(* Logix 5000 Rung export; software revision 16.03 *)

MODULES
   Local : vendor None type None code None
   PDPMV1_LEGACY : vendor None type None code None
END_MODULES

TYPE PDPMV1_SetSlaveAddress_In :   // Mailbox response
STRUCT
   ByteCount : INT;   // Byte count data block
   NewSlaveAddress : SINT;   // Range 1 to 125, specifies the new address of the slave.
   CurrentSlaveAddress : SINT;   // Range 1 to 125, specifies the current address of the slave.
   SlaveIdentNumber : INT;   // Ident number for the slave, which address should be altered.
   No_add_Chg : INT;   // This parameter specifies whether it is allowed to change the slave address again
   ErrorCode1_2 : INT;   // If other than 0, refer to user manual for code information
   ErrorCode3_4 : INT;   // If other than 0, refer to user manual for code information
   ReturnCode : INT;   // If other than 0, refer to user manual for code information
   FaultInformation : INT;   // If other than 0, refer to user manual for code information
   MessageDataByte : SINT[400];   // Message data byte array for user-specific data
END_STRUCT
END_TYPE

TYPE PDPMV1_Module :   // Status data
STRUCT
   Mod_scan_count : INT;   // Incremented every module scan loop
   Mod_output_update : INT;   // Incremented at every output scan
   Mod_input_update : INT;   // Incremented at every input scan
   Mod_out_MB : INT;   // Incremented at every output mailbox processing
   Mod_in_MB : INT;   // Incremented at every intput mailbox processing
   Mod_alarm_ind : INT;   // Incremented at every alarm indication
   Mod_alarm_con : INT;   // Incremented at every alarm confirmation
   Reserved1 : INT;   // Reserved
   Reserved2 : INT;   // Reserved
END_STRUCT
END_TYPE

TYPE PDPMV1_GetSlaveConfig :   // GetSlaveConfig mailobox to retrieve configuration data from specific PROFIBUS slaves
STRUCT
   Out : PDPMV1_GetSlaveConfig_Out;   // mailbox request
   In : PDPMV1_GetSlaveConfig_In;   // mailbox response
END_STRUCT
END_TYPE

TYPE PDPMV1_CRC :   // Module CRC status
STRUCT
   ProfibusCRC : DINT;   // CRC value related to the PROFIBUS configuration that was downloaded to the module
   ModuleCRC : DINT;   // CRC value related to the module configuration that was downloaded to the module
END_STRUCT
END_TYPE

TYPE PDPMV1_backplane2 :   // Stores variables used by sample ladder logic for handshaking purposes.
STRUCT
   LastRead : INT;   // Last read block index received from the module
   LastWrite : INT;   // Last write block index received from the module
   BlockIndex : INT;   // Block index of each copy of PROFIBUS input and output blocks
END_STRUCT
END_TYPE

TYPE PDPMV1_SetSlaveMode_Out :   // Mailbox Request
STRUCT
   GroupSelect : SINT;   // Range 01h to FFh (Bit Coded). This parameter determines which group to address. Refer to the user manual for examples
   SlaveAddress : SINT;   // Range 1 to 125; 127 (Multicast address).
   ControlCommand : PDPMV1_ControlCommand;   // This parameter specifies the command to send (Unsync/Sync and Unfreeze/Freeze).
END_STRUCT
END_TYPE

TYPE PDPMV1_StopSlaves_Out :   // Mailbox request
STRUCT
   SlaveNumber : SINT[126];   // Slave number designation (1-125)
END_STRUCT
END_TYPE

TYPE PDPMV1_GetSlaveConfig_Out :   // GetSlaveConfig mailbox request
STRUCT
   SlaveAddress : INT;   // Destination of slave (1-125)
END_STRUCT
END_TYPE

TYPE PDPMV1_GetSlaveDiagnostics_In :   // GetSlaveDiagnostics mailbox response
STRUCT
   SlaveAddress : INT;   // Destination of slave (1-125)
   ExtendedFaultInfo : INT;   // If other than 0, refer to user manual for code information
   FaultInformation : INT;   // If other than 0, refer to user manual for code information
   StationStatus1_2 : INT;   // Status of station types 1 and 2
   StationStatus3_4 : INT;   // Status of station types 3 and 4
   IdentNumber : INT;   // Unique ID assigned by the PROFIBUS User Organization
   ExtendedDiagnosticData : INT[200];   // Slave user-specific data. Refer to actual slave documentation for info
END_STRUCT
END_TYPE

TYPE PDPMV1_AcyclicRead :   // DPV1 acyclic read mailbox data structure
STRUCT
   Out : PDPMV1_AcyclicRead_Out;   // mailbox request
   In : PDPMV1_AcyclicRead_In;   // mailbox response
END_STRUCT
END_TYPE

TYPE PDPMV1_StartSlaves_In :   // Mailbox Response
STRUCT
   AdditionalFaultInfo : INT;   // If other than 0, refer to user manual for code information
   FaultInformation : INT;   // If other than 0, refer to user manual for code information
   SlaveNumber : SINT[126];   // Slave number designation (1-125)
END_STRUCT
END_TYPE

TYPE PDPMV1_AcyclicWrite :   // DPV1 acyclic write mailbox data structure
STRUCT
   Out : PDPMV1_AcyclicWrite_Out;   // Mailbox request
   In : PDPMV1_AcyclicWrite_In;   // Mailbox response
END_STRUCT
END_TYPE

TYPE PDPMV1_StartSlaves_Out :   // Mailbox Request
STRUCT
   SlaveNumber : SINT[126];   // Slave number designation (1-125)
END_STRUCT
END_TYPE

TYPE PDPMV1_GetSlaveDiagnostics :   // GetSlaveDiagnostics mailbox to retrieve diagnostic information from specific PROFIBUS slaves
STRUCT
   Out : PDPMV1_GetSlaveDiagnostics_Out;   // Mailbox request
   In : PDPMV1_GetSlaveDiagnostics_In;   // Mailbox response
END_STRUCT
END_TYPE

TYPE PDPMV1_backplane :   // Stores variables used by sample ladder logic for handshaking purposes.
STRUCT
   Read : INT;   // Backplane read statistics
   Write : INT;   // Backplane write statistics
   Error : INT;   // Backplane error statistics
   LastRead : INT;   // Last read block index received from the module
   LastWrite : INT;   // Last write block index received from the module
   BlockIndex : INT;   // Block index of each copy of PROFIBUS input and output blocks
END_STRUCT
END_TYPE

TYPE PDPMV1_other_status :
STRUCT
   Cfg_file_error : INT;   // Bit0 = PDPMV1.CFG, Bit 1 = WATTCP.CFG, Bit 2 = PDPMV1.DDB, Bit3=PDPMV1.XML
   R_120 : INT;   // Not Used
   R_122 : INT;   // Not Used
   R_124 : INT;   // Not Used
   R_126 : INT;   // Not Used
   R_128 : INT;   // Not Used
   R_130 : INT;   // Not Used
   R_132 : INT;   // Not Used
   R_134 : INT;   // Not Used
   R_136 : INT;   // Not Used
   R_138 : INT;   // Not Used
   R_140 : INT;   // Not Used
   R_142 : INT;   // Not Used
   R_144 : INT;   // Not Used
   In_MB_queue : INT;   // Number of messages in the input mailbox queue
   Out_MB_queue : INT;   // Number of messages in the output mailbox queue
   Alarm_MB_queue : INT;   // Number of messages in the alarm mailbox queue
   Last_out_MB : INT;   // Number of messages in the output mailbox queue
   Cur_in_MB : INT;   // Number of messages currently in the input mailbox queue
   Cur_alarm_MB : INT;   // Number of messages currently in the alarm mailbox queue
END_STRUCT
END_TYPE

TYPE PDPMV1_ControlCommand :   // Option bits for SetSlaveMode mailbox
STRUCT
   Reserved1 : BOOL;   // Reserved
   Reserved2 : BOOL;   // Reserved
   Unfreeze_Input : BOOL;   // Freeze mode is concluded when initiated
   Freeze_Input : BOOL;   // Causes the addressed slave to assume freeze mode.
   Unsynchronize_Output : BOOL;   // Unsynchronized output data
   Synchronize_Output : BOOL;   // Synchronized output data
   Reserved3 : BOOL[32];   // Reserved
END_STRUCT
END_TYPE

TYPE PDPMV1_AcyclicWrite_In :   // DPV1 acyclic write mailbox response
STRUCT
   ByteCount : INT;   // Byte count data block
   SlotNumber : SINT;   // Used in the slave to address the desired data block.
   SlaveAddress : SINT;   // Destination of slave (1-125)
   Length : SINT;   // Specifies the number of bytes of the data block to read
   Index : SINT;   // Index block
   ErrorDecode : SINT;   // If other than 0, refer to user manual for code information
   ErrorCode2 : SINT;   // If other than 0, refer to user manual for code information
   ErrorCode1 : SINT;   // If other than 0, refer to user manual for code information
   ExtendedFaultInfo : INT;   // If other than 0, refer to user manual for code information
   FaultInformation : INT;   // If other than 0, refer to user manual for code information
   Data : SINT[200];   // Returned data [1...n] array
END_STRUCT
END_TYPE

TYPE PDPMV1_AcyclicRead_Out :   // DPV1 acyclic read mailbox request
STRUCT
   SlotNumber : SINT;   // Used in the slave to address the desired data block.
   SlaveAddress : SINT;   // Destination of slave (1-125)
   Length : SINT;   // Specifies the number of bytes of the data block to read
   Index : SINT;   // Index block
END_STRUCT
END_TYPE

TYPE PDPMV1_Fieldbus :   // Fieldbus status
STRUCT
   FB_Slave_Cfg_List : SINT[16];   // Bitmap structure containing PROFIBUS slave configuration (bit x = 1 means slave x is configured)
   FB_Slave_Data_xfer : SINT[16];   // Bitmap structure containing PROFIBUS slave data exchange status (bit x = 1 means slave x is transferring data to the module)
   FB_Slave_Diag : SINT[16];   // Bitmap structure containing PROFIBUS slave diagnostic info (bit x = 1 means slave x is reporting diagnostics)
   FB_Pad_Byte : SINT;   // Reserved
   FB_op_state : SINT;   // Operation state ( 00 = offline, 40 = stop, 80 = clear, C0= operate)
   FB_ident_MSB : SINT;   // Master identification code (most significant byte)
   FB_ident_LSB : SINT;   // Master identification code (least significant byte)
END_STRUCT
END_TYPE

TYPE PDPMV1_StopSlaves_In :   // Mailbox response
STRUCT
   AdditionalFaultinfo : INT;   // If other than 0, refer to user manual for code information
   FaultInformation : INT;   // If other than 0, refer to user manual for code information
   SlaveNumber : SINT[126];   // Slave number designation (1-125)
END_STRUCT
END_TYPE

TYPE PDPMV1_StartSlaves :   // StartSlaves mailbox allows the processor to restart communication to slaves that were previoulsy interrupted by StopSlaves
STRUCT
   Out : PDPMV1_StartSlaves_Out;   // Mailbox Request
   In : PDPMV1_StartSlaves_In;   // Mailbox Response
END_STRUCT
END_TYPE

TYPE PDPMV1_SetSlaveMode :   // SetSlaveMode mailbox that allows the processor to change the slave mode to interrupt input or output data update
STRUCT
   Out : PDPMV1_SetSlaveMode_Out;   // Mailbox Request
   In : PDPMV1_SetSlaveMode_In;   // Mailbox Response
END_STRUCT
END_TYPE

TYPE PDPMV1_Mailbox :   // Stores all mailbox request and response registers
STRUCT
   GetLiveList : PDPMV1_GetLiveList;   // This command returns 127 bytes of information about the nodes on the network.
   GetSlaveConfig : PDPMV1_GetSlaveConfig;   // This command reads the actual configuration (identifier bytes) of a specified slave.
   SetSlaveMode : PDPMV1_SetSlaveMode;   // This control command is transmitted as multicast commands.
   GetSlaveDiagnostics : PDPMV1_GetSlaveDiagnostics;   // This command reads diagnostic data from a specified slave.
   SetSlaveAddress : PDPMV1_SetSlaveAddress;   // This command makes it possible to set the node address of a specified slave, if the slave supports this feature.
   StartSlaves : PDPMV1_StartSlaves;   // This mailbox message starts a selection of slaves that was previously removed from the processing cycle by means of the mailbox
   StopSlaves : PDPMV1_StopSlaves;   // This mailbox message stops a selection of slaves from the processing cycle.
   AcyclicRead : PDPMV1_AcyclicRead;   // This encapsulates a DPV1 Class 1 acyclic read request.
   AcyclicWrite : PDPMV1_AcyclicWrite;   // This encapsulates a DPV1 Class 1 acyclic write request.
   Alarm : PDPMV1_Alarm;   // This indicates to the application that a DPV1 slave has transferred an Alarm message to the master.
END_STRUCT
END_TYPE

TYPE PDPMV1_AcyclicWrite_Out :   // DPV1 acyclic write mailbox request
STRUCT
   SlotNumber : SINT;   // Used in the slave to address the desired data block.
   SlaveAddress : SINT;   // Destination of slave (1-125)
   Length : SINT;   // Specifies the number of bytes of the data block to read
   Index : SINT;   // Index block
   Data : SINT[200];   // Data that should be written [1...n]
END_STRUCT
END_TYPE

TYPE PDPMV1_ModuleDef :   // Main module definition
STRUCT
   Output : SINT[1536];   // Output data
   Input : SINT[1536];   // Input data
   BP : PDPMV1_backplane2;   // Backplane status
   Status : PDPMV1_Status;   // Module status information
   MailboxCommand : PDPMV1_Command;   // Mailbox Command
   Mailbox : PDPMV1_Mailbox;   // Mailbox tags for optional applications
   CRC : PDPMV1_CRC_Struct;   // CRC status
   MailboxControl : PDPMV1_MBControl;   // Mailbox Control
   Util : PDPMV1_Util;   // Internal tags used for ladder logic processing. User applications should not overwrite any Util tags
END_STRUCT
END_TYPE

TYPE PDPMV1_Util :
STRUCT
   ByteSwapUtil : INT;   // Used for byte swap logic
   TempInt : INT;   // Used for integer formatting
END_STRUCT
END_TYPE

TYPE PDPMV1_GetLiveList :   // GetLiveList mailbox to retrieve the live list information from PROFIBUS network, informing the slaves that are communicating
STRUCT
   ReturnCode : SINT;   // Returned code about the nodes on the network
   FaultInfo : SINT;   // If other than 0, refer to user manual for code information
   Station : SINT[127];   // Station type contents.
END_STRUCT
END_TYPE

TYPE PDPMV1_MBControl :   // PDPMV1 MBControl status.
STRUCT
   Out_MB_index : INT;   // Reserved
   In_MB_index : INT;   // Reserved
   Alarm_MB_index : INT;   // Reserved
   In_Last_Out_MB : INT;   // Last out mailbox message ID processed from output image
   In_Last_In_MB : INT;   // Current in mailbox control index
   In_Last_Alarm_MB : INT;   // Current alarm control index
END_STRUCT
END_TYPE

TYPE PDPMV1_SetSlaveMode_In :   // Mailbox response
STRUCT
   GroupSelect : SINT;   // Range 01h to FFh (Bit Coded). This parameter determines which group to address. Refer to the user manual for examples
   SlaveAddress : SINT;   // Range 1 to 125; 127 (Multicast address).
   ControlCommand : PDPMV1_ControlCommand;   // This parameter specifies the command to send (Unsync/Sync and Unfreeze/Freeze).
   ExtendedFaultInfo : INT;   // If other than 0, refer to user manual for code information
   FaultInformation : INT;   // If other than 0, refer to user manual for code information
END_STRUCT
END_TYPE

TYPE PDPMV1_Status :   // Status data from the MVI56-PDPMV1 module
STRUCT
   Pattern : SINT[12];   // Module indentification code
   Input_Size : INT;   // Configured PROFIBUS input data size
   Output_Size : INT;   // Configured PROFIBUS output data size
   Reserved_16 : INT;   // Not Used
   Reserved_18 : INT;   // Not Used
   Reserved_20 : INT;   // Not Used
   Input_Swap : SINT;   // Configured input swap byte option (1=swap bytes, 0= no swap)
   Output_Swap : SINT;   // Configured output swap byte option (1=swap bytes, 0= no swap)
   Module_Major_Ver : SINT;   // Module major firmware version
   Module_Minor_Ver : SINT;   // Module minor firmware version
   Fieldbus : PDPMV1_Fieldbus;   // PROFIBUS network status information
   Control : PDPMV1_Control;   // Module information
   Profibus_CRC32 : DINT;   // CRC value related to the PROFIBUS configuration that was downloaded to the module
   Module_CRC32 : DINT;   // CRC value related to the module configuration that was downloaded to the module
   Module : PDPMV1_Module;   // General module status to monitor data, mailbox and alarm exchange between the processor and the module
   Backplane : PDPMV1_backplane;   // Backplane status information
   Other : PDPMV1_other_status;   // General mailbox and cfg error information
END_STRUCT
END_TYPE

TYPE PDPMV1_SetSlaveAddress :   // SetSlaveAddress mailbox that allows the module to dynamically change a PRIDUBUS address (only for slaves that supports it)
STRUCT
   Out : PDPMV1_SetSlaveAddress_Out;   // Mailbox request
   In : PDPMV1_SetSlaveAddress_In;   // Mailbox response
END_STRUCT
END_TYPE

TYPE PDPMV1_AcyclicRead_In :   // DPV1 acyclic read mailbox response
STRUCT
   ByteCount : INT;   // Byte count data block
   SlotNumber : SINT;   // Used in the slave to address the desired data block.
   SlaveAddress : SINT;   // Destination of slave (1-125)
   Length : SINT;   // Specifies the number of bytes of the data block to read
   Index : SINT;   // Index block
   ErrorDecode : SINT;   // If other than 0, refer to user manual for code information
   ErrorCode2 : SINT;   // If other than 0, refer to user manual for code information
   ErrorCode1 : SINT;   // If other than 0, refer to user manual for code information
   ExtendedFaultInfo : INT;   // If other than 0, refer to user manual for code information
   FaultInformation : INT;   // If other than 0, refer to user manual for code information
   Data : SINT[200];   // Returned data [1...n] array
END_STRUCT
END_TYPE

TYPE PDPMV1_StopSlaves :   // StopSlaves mailbox allows the processor to interrupt communication to specific PROFIBUS slaves
STRUCT
   Out : PDPMV1_StopSlaves_Out;   // Mailbox Request
   In : PDPMV1_StopSlaves_In;   // Mailbox Response
END_STRUCT
END_TYPE

TYPE PDPMV1_SetSlaveAddress_Out :   // Mailbox request
STRUCT
   ByteCount : INT;   // Byte count data block
   NewSlaveAddress : SINT;   // Range 1 to 125, specifies the new address of the slave.
   CurrentSlaveAddress : SINT;   // Range 1 to 125, specifies the current address of the slave.
   SlaveIdentNumber : INT;   // Ident number for the slave, which address should be altered.
   No_add_Chg : INT;   // This parameter specifies whether it is allowed to change the slave address again
   MessageDataByte : SINT[400];   // Message data byte array for user-specific data
END_STRUCT
END_TYPE

TYPE PDPMV1_GetSlaveConfig_In :   // GetSlaveConfig mailbox response
STRUCT
   ByteCount : INT;   // Byte count data block
   WordCount : INT;   // Word count data block
   SlaveAddress : INT;   // Destination of slave (1-125)
   ErrorCode : INT[1];   // If other than 0, refer to user manual for code information
   ReturnCode : INT;   // If other than 0, refer to user manual for code information
   FaultInformation : INT;   // If other than 0, refer to user manual for code information
   Identifier : SINT[245];   // Configuration from a specific connected PROFIBUS slave
END_STRUCT
END_TYPE

TYPE PDPMV1_GetSlaveDiagnostics_Out :   // GetSlaveDiagnostics mailbox request
STRUCT
   SlaveAddress : INT;   // Destination of slave (1-125)
END_STRUCT
END_TYPE

TYPE PDPMV1_Command :   // This data structure contains the command bits to request mailbox, retrieve status from the module
STRUCT
   StopMode : BOOL;   // Set the module to stop mode (PROFIBUS communication is interrupted in stop mode)
   OperateMode : BOOL;   // Set the module to operate mode (module only communicates through PROFIBUS)
   ClearMode : BOOL;   // Set the module to clear mode (outputs are disabled)
   SynchCRC : BOOL;   // CRC synchronization
   GetLiveList : BOOL;   // Request the Live List information from the module
   GetSlaveConfig : BOOL;   // Request configuration information from a slave
   SetSlaveMode : BOOL;   // Set the module to stop mode (PROFIBUS communication is interrupted in stop mode)
   GetSlaveDiagnostics : BOOL;   // Requests slave diagnostics from a slave
   SetSlaveAddress : BOOL;   // Change the slave's PROFIBUS address (only if slave supports this feature)
   StartSlaves : BOOL;   // Restarts PROFIBUS communication with one or more slaves after a "StopSlave" mailbox
   StopSlaves : BOOL;   // Stop PROFIBUS communication with one or more slaves
   AcyclicRead : BOOL;   // Request the module to send acyclic read message to slave
   AcyclicWrite : BOOL;   // Request the module to send acyclic write message to slave
END_STRUCT
END_TYPE

TYPE PDPMV1_Alarm :   // DPV1 alarm data received by the module
STRUCT
   ByteCount : INT;   // Byte count data block
   SlotNumber : SINT;   // Used in the slave to address the desired data block. Range 0-254
   SlaveAddress : SINT;   // Destination of slave (1-125)
   AlarmSpecAck : SINT;   // Additional alarm information
   SeqNumber : SINT;   // Unique ID number of the alarm. Range 0-31
   ExtDiag : SINT;   // Extended Diagnostic Flag (FFh - flag set and 00h - flag cleared).
   AlarmType : SINT;   // Identifies alarm type. Range is from 1 to 6, 32 to 126.
   FaultInformation : INT;   // If other than 0, refer to user manual for code information
   Data : SINT[500];   // Returned data [1...n] array with additional manf. spec alarm info.
END_STRUCT
END_TYPE

TYPE PDPMV1_Control :   // Control status
STRUCT
   serial_number : SINT[4];   // Module serial number
   version_MSB : SINT;   // Module version number (most significant byte)
   version_LSB : SINT;   // Module version number (least significant byte)
   mod_status_MSB : SINT;   // Module status (most significant byte)
   mod_status_LSB : SINT;   // Module status (least significant byte)
END_STRUCT
END_TYPE

TYPE PDPMV1_CRC_Struct :   // Module CRC structures
STRUCT
   In : PDPMV1_CRC;   // Mailbox response
   Out : PDPMV1_CRC;   // Mailbox request
END_STRUCT
END_TYPE

ADD_ON_INSTRUCTION AOI56PDPMV1_LEGACY   (* revision 1.4, vendor Prosoft Technology Inc., ExecutePrescan *)
// Add-On for MVI56-PDPMV1 (Legacy) module.
// Revision note:
// v1.4 - AOI generated a minor fault in the CPU due to an arithmetic overflow, modified user defined data type Acyclic read/write
VAR_IN_OUT
   Connection_Input : INT[250]; {required}   // Connection input to be associated to the MVI56PDPMV1 input array
   Connection_Output : INT[248]; {required}   // Connection output to be associated to the MVI56PDPMV1 output array
   MVI56PDPMV1 : PDPMV1_ModuleDef; {required}   // Main module controller tag
END_VAR
VAR
   MJFAULTS : DINT[12];   // power up handling
END_VAR

ROUTINE Logic   (* ladder *)
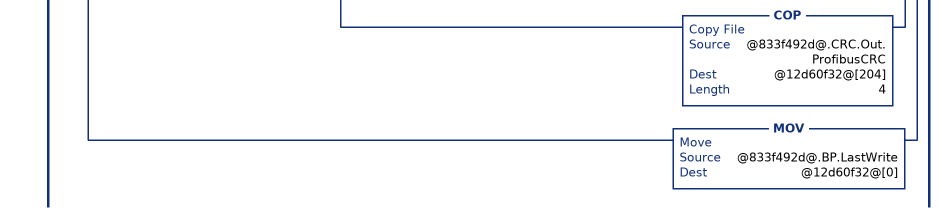
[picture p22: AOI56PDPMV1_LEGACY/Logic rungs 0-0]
   // This rung updates the variable that is used to store the latest Block ID sent by the module
   0: NEQ(@1acd65bb@[249],@833f492d@.BP.LastRead)[MOV(@1acd65bb@[249],@833f492d@.BP.LastRead) ,[EQU(@833f492d@.BP.LastRead,-1) ,EQU(@833f492d@.BP.LastRead,0) ] [COP(@1acd65bb@[0],@833f492d@.Status.Pattern[0],16) ,COP(@1acd65bb@[11],@833f492d@.Status.Input_Swap,4) ,COP(@1acd65bb@[13],@833f492d@.Status.Fieldbus.FB_Slave_Cfg_List[0],52) ,COP(@1acd65bb@[39],@833f492d@.Status.Control.serial_number[0],8) ,COP(@1acd65bb@[43],@833f492d@.Status.Profibus_CRC32,2) ,COP(@1acd65bb@[47],@833f492d@.Status.Module.Mod_scan_count,9) ,COP(@1acd65bb@[56],@833f492d@.Status.Backplane.Read,3) ,COP(@1acd65bb@[59],@833f492d@.Status.Other.Cfg_file_error,20) ] ,LIM(1,@833f492d@.BP.LastRead,4) [CPT(@833f492d@.BP.BlockIndex,(@833f492d@.BP.LastRead-1)*400) ,LIM(1,@833f492d@.BP.LastRead,3) COP(@1acd65bb@[0],@833f492d@.Input[@833f492d@.BP.BlockIndex],400) ,EQU(@833f492d@.BP.LastRead,4) COP(@1acd65bb@[0],@833f492d@.Input[1200],336) ,COP(@1acd65bb@[200],@833f492d@.MailboxControl.In_Last_Out_MB,3) ,COP(@1acd65bb@[204],@833f492d@.CRC.In.ProfibusCRC,2) ] ,LIM(100,@833f492d@.BP.LastRead,109) [EQU(@1acd65bb@[2],24) COP(@1acd65bb@[16],@833f492d@.Mailbox.GetLiveList.Station[0],127) ,EQU(@1acd65bb@[2],3) [COP(@1acd65bb@[8],@833f492d@.Mailbox.SetSlaveMode.In.GroupSelect,2) ,MOV(@1acd65bb@[9],@833f492d@.Util.TempInt) ,SWPB(@833f492d@.Util.TempInt,REVERSE,@833f492d@.Util.ByteSwapUtil) ,COP(@833f492d@.Util.ByteSwapUtil,@833f492d@.Mailbox.SetSlaveMode.In.ControlCommand,1) ,MOV(@1acd65bb@[14],@833f492d@.Mailbox.SetSlaveMode.In.ExtendedFaultInfo) ,MOV(@1acd65bb@[15],@833f492d@.Mailbox.SetSlaveMode.In.FaultInformation) ] ,EQU(@1acd65bb@[2],4) [MOV(@1acd65bb@[8],@833f492d@.Util.ByteSwapUtil) ,SWPB(@833f492d@.Util.ByteSwapUtil,REVERSE,@833f492d@.Mailbox.GetSlaveDiagnostics.In.SlaveAddress) ,MOV(@1acd65bb@[14],@833f492d@.Mailbox.GetSlaveDiagnostics.In.ExtendedFaultInfo) ,MOV(@1acd65bb@[15],@833f492d@.Mailbox.GetSlaveDiagnostics.In.FaultInformation) ,MOV(@1acd65bb@[16],@833f492d@.Mailbox.GetSlaveDiagnostics.In.StationStatus1_2) ,MOV(@1acd65bb@[17],@833f492d@.Mailbox.GetSlaveDiagnostics.In.StationStatus3_4) ,MOV(@1acd65bb@[18],@833f492d@.Mailbox.GetSlaveDiagnostics.In.IdentNumber) ,COP(@1acd65bb@[19],@833f492d@.Mailbox.GetSlaveDiagnostics.In.ExtendedDiagnosticData[0],200) ] ,EQU(@1acd65bb@[2],5) [MOV(@1acd65bb@[3],@833f492d@.Mailbox.GetSlaveConfig.In.ByteCount) ,MOV(@1acd65bb@[8],@833f492d@.Util.ByteSwapUtil) ,SWPB(@833f492d@.Util.ByteSwapUtil,REVERSE,@833f492d@.Mailbox.GetSlaveConfig.In.SlaveAddress) ,COP(@1acd65bb@[12],@833f492d@.Mailbox.GetSlaveConfig.In.ErrorCode[0],2) ,MOV(@1acd65bb@[14],@833f492d@.Mailbox.GetSlaveConfig.In.ReturnCode) ,MOV(@1acd65bb@[15],@833f492d@.Mailbox.GetSlaveConfig.In.FaultInformation) ,COP(@1acd65bb@[16],@833f492d@.Mailbox.GetSlaveConfig.In.Identifier[0],@833f492d@.Mailbox.GetSlaveConfig.In.ByteCount) ] ,EQU(@1acd65bb@[2],6) [MOV(@1acd65bb@[3],@833f492d@.Mailbox.SetSlaveAddress.In.ByteCount) ,COP(@1acd65bb@[8],@833f492d@.Mailbox.SetSlaveAddress.In.NewSlaveAddress,2) ,MOV(@1acd65bb@[9],@833f492d@.Mailbox.SetSlaveAddress.In.SlaveIdentNumber) ,MOV(@1acd65bb@[10],@833f492d@.Util.ByteSwapUtil) ,SWPB(@833f492d@.Util.ByteSwapUtil,REVERSE,@833f492d@.Mailbox.SetSlaveAddress.In.No_add_Chg) ,MOV(@1acd65bb@[12],@833f492d@.Mailbox.SetSlaveAddress.In.ErrorCode1_2) ,MOV(@1acd65bb@[13],@833f492d@.Mailbox.SetSlaveAddress.In.ErrorCode3_4) ,MOV(@1acd65bb@[14],@833f492d@.Mailbox.SetSlaveAddress.In.ReturnCode) ,MOV(@1acd65bb@[15],@833f492d@.Mailbox.SetSlaveAddress.In.FaultInformation) ,COP(@1acd65bb@[16],@833f492d@.Mailbox.SetSlaveAddress.In.MessageDataByte[0],@833f492d@.Mailbox.SetSlaveAddress.In.ByteCount) ] ,EQU(@1acd65bb@[2],11) [MOV(@1acd65bb@[14],@833f492d@.Mailbox.StartSlaves.In.AdditionalFaultInfo) ,MOV(@1acd65bb@[15],@833f492d@.Mailbox.StartSlaves.In.FaultInformation) ,COP(@1acd65bb@[16],@833f492d@.Mailbox.StartSlaves.In.SlaveNumber[0],126) ] ,EQU(@1acd65bb@[2],12) [MOV(@1acd65bb@[14],@833f492d@.Mailbox.StopSlaves.In.AdditionalFaultinfo) ,MOV(@1acd65bb@[15],@833f492d@.Mailbox.StopSlaves.In.FaultInformation) ,COP(@1acd65bb@[16],@833f492d@.Mailbox.StopSlaves.In.SlaveNumber[0],126) ] ,EQU(@1acd65bb@[2],32) [MOV(@1acd65bb@[3],@833f492d@.Mailbox.AcyclicRead.In.ByteCount) ,COP(@1acd65bb@[8],@833f492d@.Mailbox.AcyclicRead.In.SlotNumber,2) ,COP(@1acd65bb@[9],@833f492d@.Mailbox.AcyclicRead.In.Length,2) ,COP(@1acd65bb@[12],@833f492d@.Mailbox.AcyclicRead.In.ErrorDecode,1) ,COP(@1acd65bb@[13],@833f492d@.Mailbox.AcyclicRead.In.ErrorCode2,2) ,MOV(@1acd65bb@[14],@833f492d@.Mailbox.AcyclicRead.In.ExtendedFaultInfo) ,MOV(@1acd65bb@[15],@833f492d@.Mailbox.AcyclicRead.In.FaultInformation) ,COP(@1acd65bb@[16],@833f492d@.Mailbox.AcyclicRead.In.Data[0],@833f492d@.Mailbox.AcyclicRead.In.ByteCount) ] ,EQU(@1acd65bb@[2],33) [MOV(@1acd65bb@[3],@833f492d@.Mailbox.AcyclicWrite.In.ByteCount) ,COP(@1acd65bb@[8],@833f492d@.Mailbox.AcyclicWrite.In.SlotNumber,2) ,COP(@1acd65bb@[9],@833f492d@.Mailbox.AcyclicWrite.In.Length,2) ,COP(@1acd65bb@[12],@833f492d@.Mailbox.AcyclicWrite.In.ErrorDecode,1) ,COP(@1acd65bb@[13],@833f492d@.Mailbox.AcyclicWrite.In.ErrorCode2,2) ,MOV(@1acd65bb@[14],@833f492d@.Mailbox.AcyclicWrite.In.ExtendedFaultInfo) ,MOV(@1acd65bb@[15],@833f492d@.Mailbox.AcyclicWrite.In.FaultInformation) ,COP(@1acd65bb@[16],@833f492d@.Mailbox.AcyclicWrite.In.Data[0],@833f492d@.Mailbox.AcyclicWrite.In.ByteCount) ] ] ,LIM(200,@833f492d@.BP.LastRead,209) [MOV(@1acd65bb@[3],@833f492d@.Mailbox.Alarm.ByteCount) ,COP(@1acd65bb@[8],@833f492d@.Mailbox.Alarm.SlotNumber,2) ,COP(@1acd65bb@[9],@833f492d@.Mailbox.Alarm.AlarmSpecAck,2) ,COP(@1acd65bb@[10],@833f492d@.Mailbox.Alarm.ExtDiag,2) ,MOV(@1acd65bb@[15],@833f492d@.Mailbox.Alarm.FaultInformation) ,COP(@1acd65bb@[16],@833f492d@.Mailbox.Alarm.Data[0],@833f492d@.Mailbox.Alarm.ByteCount) ] ,MOV(@1acd65bb@[248],@833f492d@.BP.LastWrite) ,XIC(@833f492d@.MailboxCommand.StopMode) [MOV(100,@833f492d@.BP.LastWrite) ,MOV(2,@12d60f32@[1]) ,MOV(16386,@12d60f32@[2]) ,MOV(2,@12d60f32@[3]) ,MOV(0,@12d60f32@[4]) ,MOV(1,@12d60f32@[5]) ,MOV(1,@12d60f32@[6]) ,MOV(0,@12d60f32@[7]) ,MOV(0,@12d60f32@[8]) ,MOV(16384,@12d60f32@[9]) ,OTU(@833f492d@.MailboxCommand.StopMode) ] ,XIC(@833f492d@.MailboxCommand.OperateMode) [MOV(101,@833f492d@.BP.LastWrite) ,MOV(1,@12d60f32@[1]) ,MOV(16386,@12d60f32@[2]) ,MOV(2,@12d60f32@[3]) ,MOV(0,@12d60f32@[4]) ,MOV(1,@12d60f32@[5]) ,MOV(1,@12d60f32@[6]) ,MOV(0,@12d60f32@[7]) ,MOV(0,@12d60f32@[8]) ,MOV(-16384,@12d60f32@[9]) ,OTU(@833f492d@.MailboxCommand.OperateMode) ] ,XIC(@833f492d@.MailboxCommand.ClearMode) [MOV(102,@833f492d@.BP.LastWrite) ,MOV(3,@12d60f32@[1]) ,MOV(16386,@12d60f32@[2]) ,MOV(2,@12d60f32@[3]) ,MOV(0,@12d60f32@[4]) ,MOV(1,@12d60f32@[5]) ,MOV(1,@12d60f32@[6]) ,MOV(0,@12d60f32@[7]) ,MOV(0,@12d60f32@[8]) ,MOV(-32768,@12d60f32@[9]) ,OTU(@833f492d@.MailboxCommand.ClearMode) ] ,XIC(@833f492d@.MailboxCommand.GetLiveList) [MOV(103,@833f492d@.BP.LastWrite) ,MOV(4,@12d60f32@[1]) ,MOV(16386,@12d60f32@[2]) ,MOV(24,@12d60f32@[3]) ,MOV(0,@12d60f32@[4]) ,MOV(1,@12d60f32@[5]) ,MOV(1,@12d60f32@[6]) ,MOV(0,@12d60f32@[7]) ,MOV(0,@12d60f32@[8]) ,OTU(@833f492d@.MailboxCommand.GetLiveList) ] ,XIC(@833f492d@.MailboxCommand.GetSlaveConfig) [MOV(104,@833f492d@.BP.LastWrite) ,MOV(5,@12d60f32@[1]) ,MOV(16386,@12d60f32@[2]) ,MOV(5,@12d60f32@[3]) ,MOV(0,@12d60f32@[4]) ,MOV(1,@12d60f32@[5]) ,MOV(1,@12d60f32@[6]) ,MOV(0,@12d60f32@[7]) ,MOV(0,@12d60f32@[8]) ,SWPB(@833f492d@.Mailbox.GetSlaveConfig.Out.SlaveAddress,REVERSE,@833f492d@.Util.ByteSwapUtil) ,MOV(@833f492d@.Util.ByteSwapUtil,@12d60f32@[9]) ,OTU(@833f492d@.MailboxCommand.GetSlaveConfig) ] ,XIC(@833f492d@.MailboxCommand.SetSlaveMode) [MOV(105,@833f492d@.BP.LastWrite) ,MOV(6,@12d60f32@[1]) ,MOV(16386,@12d60f32@[2]) ,MOV(3,@12d60f32@[3]) ,MOV(0,@12d60f32@[4]) ,MOV(1,@12d60f32@[5]) ,MOV(1,@12d60f32@[6]) ,MOV(0,@12d60f32@[7]) ,MOV(0,@12d60f32@[8]) ,COP(@833f492d@.Mailbox.SetSlaveMode.Out.GroupSelect,@12d60f32@[9],1) ,COP(@833f492d@.Mailbox.SetSlaveMode.Out.ControlCommand,@833f492d@.Util.TempInt,1) ,SWPB(@833f492d@.Util.TempInt,REVERSE,@833f492d@.Util.ByteSwapUtil) ,MOV(@833f492d@.Util.ByteSwapUtil,@12d60f32@[10]) ,OTU(@833f492d@.MailboxCommand.SetSlaveMode) ] ,XIC(@833f492d@.MailboxCommand.GetSlaveDiagnostics) [MOV(106,@833f492d@.BP.LastWrite) ,MOV(7,@12d60f32@[1]) ,MOV(16386,@12d60f32@[2]) ,MOV(4,@12d60f32@[3]) ,MOV(0,@12d60f32@[4]) ,MOV(1,@12d60f32@[5]) ,MOV(1,@12d60f32@[6]) ,MOV(0,@12d60f32@[7]) ,MOV(0,@12d60f32@[8]) ,SWPB(@833f492d@.Mailbox.GetSlaveDiagnostics.Out.SlaveAddress,REVERSE,@833f492d@.Util.ByteSwapUtil) ,MOV(@833f492d@.Util.ByteSwapUtil,@12d60f32@[9]) ,OTU(@833f492d@.MailboxCommand.GetSlaveDiagnostics) ] ,XIC(@833f492d@.MailboxCommand.SetSlaveAddress) [MOV(107,@833f492d@.BP.LastWrite) ,MOV(8,@12d60f32@[1]) ,MOV(16386,@12d60f32@[2]) ,MOV(6,@12d60f32@[3]) ,MOV(@833f492d@.Mailbox.SetSlaveAddress.Out.ByteCount,@12d60f32@[4]) ,MOV(1,@12d60f32@[5]) ,MOV(1,@12d60f32@[6]) ,MOV(0,@12d60f32@[7]) ,MOV(0,@12d60f32@[8]) ,COP(@833f492d@.Mailbox.SetSlaveAddress.Out.NewSlaveAddress,@12d60f32@[9],1) ,MOV(@833f492d@.Mailbox.SetSlaveAddress.Out.SlaveIdentNumber,@12d60f32@[10]) ,SWPB(@833f492d@.Mailbox.SetSlaveAddress.Out.No_add_Chg,REVERSE,@833f492d@.Util.ByteSwapUtil) ,MOV(@833f492d@.Util.ByteSwapUtil,@12d60f32@[11]) ,COP(@833f492d@.Mailbox.SetSlaveAddress.In.MessageDataByte[0],@12d60f32@[17],100) ,OTU(@833f492d@.MailboxCommand.SetSlaveAddress) ] ,XIC(@833f492d@.MailboxCommand.StartSlaves) [MOV(105,@833f492d@.BP.LastWrite) ,MOV(16,@12d60f32@[1]) ,MOV(16386,@12d60f32@[2]) ,MOV(11,@12d60f32@[3]) ,MOV(126,@12d60f32@[4]) ,MOV(1,@12d60f32@[5]) ,MOV(1,@12d60f32@[6]) ,MOV(0,@12d60f32@[7]) ,MOV(0,@12d60f32@[8]) ,MOV(0,@12d60f32@[9]) ,MOV(0,@12d60f32@[10]) ,MOV(0,@12d60f32@[11]) ,MOV(0,@12d60f32@[12]) ,MOV(0,@12d60f32@[13]) ,MOV(0,@12d60f32@[14]) ,MOV(0,@12d60f32@[15]) ,MOV(0,@12d60f32@[16]) ,COP(@833f492d@.Mailbox.StartSlaves.Out.SlaveNumber[0],@12d60f32@[17],126) ,OTU(@833f492d@.MailboxCommand.StartSlaves) ] ,XIC(@833f492d@.MailboxCommand.StopSlaves) [MOV(106,@833f492d@.BP.LastWrite) ,MOV(17,@12d60f32@[1]) ,MOV(16386,@12d60f32@[2]) ,MOV(12,@12d60f32@[3]) ,MOV(126,@12d60f32@[4]) ,MOV(1,@12d60f32@[5]) ,MOV(1,@12d60f32@[6]) ,MOV(0,@12d60f32@[7]) ,MOV(0,@12d60f32@[8]) ,MOV(0,@12d60f32@[9]) ,MOV(0,@12d60f32@[10]) ,MOV(0,@12d60f32@[11]) ,MOV(0,@12d60f32@[12]) ,MOV(0,@12d60f32@[13]) ,MOV(0,@12d60f32@[14]) ,MOV(0,@12d60f32@[15]) ,MOV(0,@12d60f32@[16]) ,COP(@833f492d@.Mailbox.StopSlaves.Out.SlaveNumber[0],@12d60f32@[17],126) ,OTU(@833f492d@.MailboxCommand.StopSlaves) ] ,XIC(@833f492d@.MailboxCommand.AcyclicRead) [MOV(108,@833f492d@.BP.LastWrite) ,MOV(9,@12d60f32@[1]) ,MOV(16386,@12d60f32@[2]) ,MOV(32,@12d60f32@[3]) ,MOV(0,@12d60f32@[4]) ,MOV(1,@12d60f32@[5]) ,MOV(1,@12d60f32@[6]) ,MOV(0,@12d60f32@[7]) ,MOV(0,@12d60f32@[8]) ,COP(@833f492d@.Mailbox.AcyclicRead.Out.SlotNumber,@12d60f32@[9],1) ,COP(@833f492d@.Mailbox.AcyclicRead.Out.Length,@12d60f32@[10],1) ,OTU(@833f492d@.MailboxCommand.AcyclicRead) ] ,XIC(@833f492d@.MailboxCommand.AcyclicWrite) [MOV(109,@833f492d@.BP.LastWrite) ,MOV(9,@12d60f32@[1]) ,MOV(16386,@12d60f32@[2]) ,MOV(33,@12d60f32@[3]) ,MOV(@833f492d@.Mailbox.AcyclicWrite.Out.Length,@12d60f32@[4]) ,MOV(1,@12d60f32@[5]) ,MOV(1,@12d60f32@[6]) ,COP(@833f492d@.Mailbox.AcyclicWrite.Out.SlotNumber,@12d60f32@[9],1) ,COP(@833f492d@.Mailbox.AcyclicWrite.Out.Length,@12d60f32@[10],1) ,COP(@833f492d@.Mailbox.AcyclicWrite.Out.Data[0],@12d60f32@[17],@833f492d@.Mailbox.AcyclicWrite.Out.Length) ,OTU(@833f492d@.MailboxCommand.AcyclicWrite) ] ,XIC(@833f492d@.MailboxCommand.SynchCRC) [MOV(@833f492d@.CRC.In.ProfibusCRC,@833f492d@.CRC.Out.ProfibusCRC) ,MOV(@833f492d@.CRC.In.ModuleCRC,@833f492d@.CRC.Out.ModuleCRC) ,OTU(@833f492d@.MailboxCommand.ClearMode) ] ,LIM(1,@833f492d@.BP.LastWrite,4) [CPT(@833f492d@.BP.BlockIndex,(@833f492d@.BP.LastWrite-1)*400) ,LIM(1,@833f492d@.BP.LastWrite,3) COP(@833f492d@.Output[@833f492d@.BP.BlockIndex],@12d60f32@[1],200) ,EQU(@833f492d@.BP.LastWrite,4) COP(@833f492d@.Output[1200],@12d60f32@[1],168) ,COP(@833f492d@.CRC.Out.ProfibusCRC,@12d60f32@[204],4) ] ,MOV(@833f492d@.BP.LastWrite,@12d60f32@[0]) ];
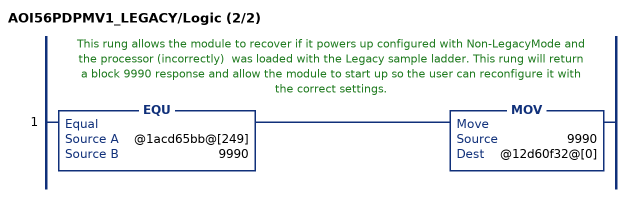
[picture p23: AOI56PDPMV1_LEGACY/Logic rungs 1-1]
   // This rung allows the module to recover if it powers up configured with Non-LegacyMode and the processor (incorrectly)  was loaded with the Legacy sample ladder. This rung will return a block 9990 response and allow the module to start up so the user can reconfigure it with the correct settings.
   1: EQU(@1acd65bb@[249],9990)MOV(9990,@12d60f32@[0]);
END_ROUTINE

ROUTINE Prescan   (* ladder *)
// PowerUp Handler
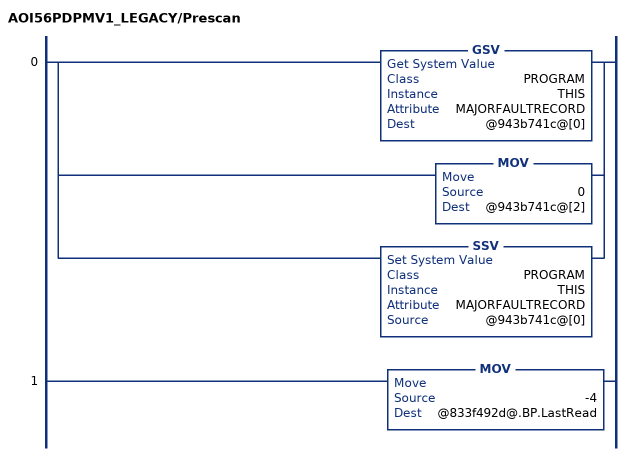
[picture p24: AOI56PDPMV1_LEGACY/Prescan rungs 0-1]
   0: [GSV(PROGRAM,THIS,MAJORFAULTRECORD,@943b741c@[0]) ,MOV(0,@943b741c@[2]) ,SSV(PROGRAM,THIS,MAJORFAULTRECORD,@943b741c@[0]) ];
   1: MOV(-4,@833f492d@.BP.LastRead);
END_ROUTINE
END_ADD_ON_INSTRUCTION

VAR_GLOBAL   (* controller tags *)
   MVI56PDPMV1 : PDPMV1_ModuleDef;
   Local:1:O : AB:1756_MODULE_INT_496Bytes:O:0;
   AOI56PDPMV1 : AOI56PDPMV1_LEGACY;
   Local:1:I : AB:1756_MODULE_INT_500Bytes:I:0;
END_VAR

PROGRAM MainProgram

ROUTINE MainRoutine   (* ladder *)
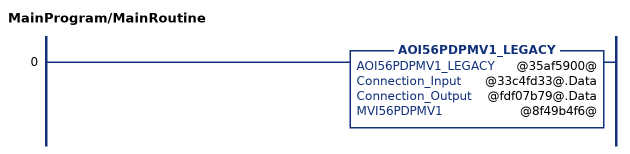
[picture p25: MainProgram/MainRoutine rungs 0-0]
   0: AOI56PDPMV1_LEGACY(@35af5900@,@33c4fd33@.Data,@fdf07b79@.Data,@8f49b4f6@);
END_ROUTINE
END_PROGRAM
